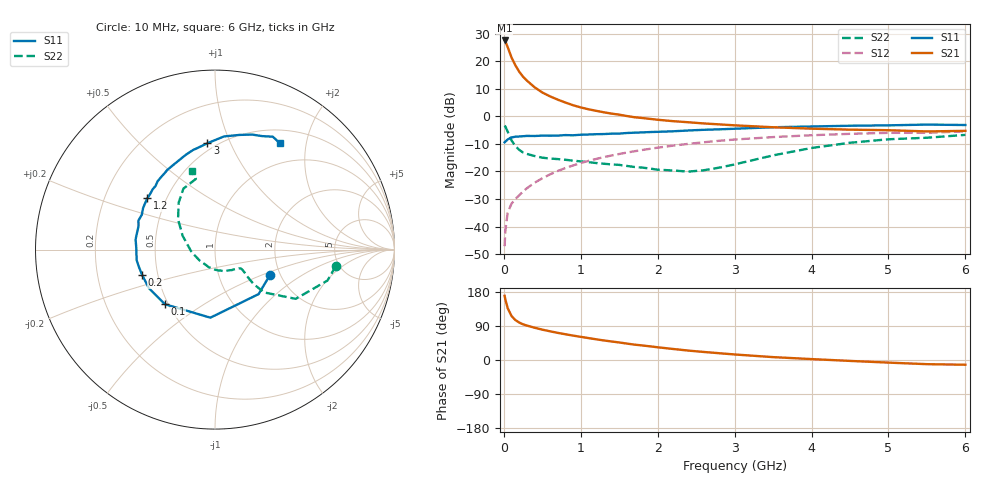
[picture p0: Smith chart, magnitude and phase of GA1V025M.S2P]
! Infineon Technologies  Discrete & RF Semiconductors
! BF775
! Si NPN RF Bipolar Junction Transistor in SOT23
! VCE = 1 V  IC = 25 mA
! Common Emitter S-Parameters:  May  1996
# GHz  S  MA  R  50
!  f  S11  S21  S12  S22
! GHz  MAG  ANG  MAG  ANG  MAG  ANG  MAG  ANG
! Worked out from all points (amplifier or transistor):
!   36 points, 10 MHz to 6 GHz, reference 50 ohm
!   highest |S21| = 27.5 dB at 10 MHz (marker M1)
!   |S21| within 3 dB of that: start of sweep to 57.68 MHz
!   unconditionally stable (mu >= 1): start of sweep to 44.5 MHz; 57.08 MHz to end of sweep
!   at 250 MHz: K = 1.73, MAG = 15.8 dB, |S12| = -27.3 dB
!   at 1.4 GHz: K = 1.79, MAG = 2.5 dB, |S12| = -14.2 dB
!   at 6 GHz: K = 1.17, MAG = -2.4 dB, |S12| = -5.5 dB
!   S11 on the Smith chart (normalised r, x): 10 MHz: 1.78, -0.56; 100 MHz: 0.48, -0.35; 200 MHz: 0.41, -0.14; 1.2 GHz: 0.39, +0.29; 3 GHz: 0.45, +0.82; 6 GHz: 0.69, +1.56
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0.01  0.3376 -24.4  23.75 169.4  0.0044 74.5  0.6795 -7.8
0.02  0.3472 -45.6  22.85 159.5  0.0085 73.7  0.6499 -15.4
0.05  0.3802 -93.9  17.97 136.7  0.0179 62.1  0.5267 -31.4
0.1  0.4128 -132.5  11.65 116.1  0.026 55.7  0.3639 -41.0
0.15  0.4265 -149.8  8.403 105.4  0.0317 56.2  0.2883 -41.8
0.2  0.4298 -160.6  6.432 98.8  0.0369 59.7  0.2456 -40.3
0.25  0.4349 -167.4  5.216 94.1  0.0432 61.3  0.2199 -38.8
0.3  0.4405 -172.4  4.436 90.8  0.0495 63.6  0.2075 -37.7
0.4  0.4388 178.6  3.356 85.2  0.0623 65.9  0.1902 -36.4
0.5  0.4459 172.8  2.701 80.1  0.075 67.1  0.1774 -36.3
0.6  0.4445 168.1  2.3 75.8  0.0882 67.4  0.1712 -37.6
0.8  0.4561 159.2  1.776 68.0  0.115 66.5  0.1625 -41.5
1.1  0.4671 146.7  1.34 57.9  0.1551 63.9  0.1474 -50.8
1.2  0.4729 142.8  1.256 54.6  0.1682 63.0  0.1418 -54.1
1.7  0.5041 126.3  0.96 40.5  0.2322 56.3  0.1202 -75.2
2.2  0.5341 112.8  0.815 29.1  0.2931 48.7  0.1039 -109.3
2.6  0.5683 102.4  0.741 21.2  0.3377 42.5  0.105 -144.5
3  0.5941 94.1  0.685 14.6  0.3783 35.9  0.1339 -176.4
3.5  0.6322 85.5  0.632 7.6  0.4195 28.0  0.1952 157.1
4.5  0.6734 72.1  0.572 -2.4  0.4804 13.3  0.3308 127.7
5.5  0.7067 62.9  0.531 -11.0  0.5009 -0.1  0.408 105.1
6  0.694 58.5  0.544 -12.5  0.5331 -4.0  0.4596 106.5
